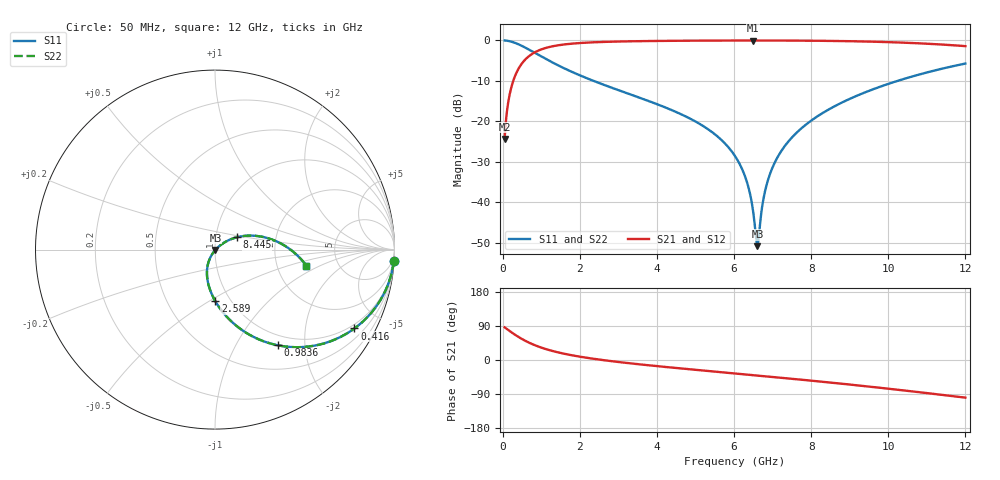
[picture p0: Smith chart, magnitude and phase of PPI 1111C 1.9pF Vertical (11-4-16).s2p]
# GHz S MA R 50
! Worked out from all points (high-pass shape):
!   1601 points, 50 MHz to 12 GHz, reference 50 ohm
!   highest |S21| = -0.03 dB at 6.496 GHz (marker M1); lowest = -24.4 dB at 50 MHz (marker M2)
!   |S21| within 3 dB of the highest: 818.2 MHz to end of sweep
!   lowest |S11| = -50.9 dB at 6.608 GHz (marker M3), VSWR 1.01, Z = 50.2 - j0.171 ohm
!   |S11| at or under -10 dB: 2.353 GHz to 10.24 GHz (7.891 GHz wide, 125 % of centre)
!   |S22| runs from -50.9 to 0.0 dB; largest |S21 - S12| = 0
!   S11 on the Smith chart (normalised r, x): 50 MHz: 1, -30; 416 MHz: 0.84, -3.62; 983.6 MHz: 0.84, -1.52; 2.589 GHz: 0.85, -0.53; 8.445 GHz: 1.26, +0.18; 12 GHz: 2.95, -0.72
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0.05  0.9982 -3.8  0.06055 86.2  0.06055 86.2  0.9982 -3.8
0.199375  0.9719 -14.9  0.2352 75.1  0.2352 75.1  0.9719 -14.9
0.4159687  0.8924 -29.5  0.4509 60.5  0.4509 60.5  0.8924 -29.5
0.6624375  0.7783 -43.2  0.6273 46.8  0.6273 46.8  0.7783 -43.2
0.9835938  0.6394 -56.6  0.768 33.4  0.768 33.4  0.6394 -56.6
1.446656  0.4889 -70.0  0.8712 19.9  0.8712 19.9  0.4889 -70.0
2.044156  0.3627 -81.8  0.9305 8.0  0.9305 8.0  0.3627 -81.8
2.589375  0.2864 -89.8  0.9565 -0.1  0.9565 -0.1  0.2864 -89.8
4.038312  0.1603 -105.8  0.9849 -16.5  0.9849 -16.5  0.1603 -105.8
5.293062  0.0817 -117.0  0.994 -28.7  0.994 -28.7  0.0817 -117.0
6.025  0.03716 -121.5  0.9964 -35.5  0.9964 -35.5  0.03716 -121.5
6.316281  0.0189 -119.9  0.9967 -38.2  0.9967 -38.2  0.0189 -119.9
6.495531  0.007667 -108.5  0.9968 -39.9  0.9968 -39.9  0.007667 -108.5
6.56275  0.003937 -84.6  0.9968 -40.5  0.9968 -40.5  0.003937 -84.6
6.607563  0.002856 -36.6  0.9968 -41.0  0.9968 -41.0  0.002856 -36.6
6.809219  0.01402 35.1  0.9966 -42.9  0.9966 -42.9  0.01402 35.1
7.033281  0.02928 39.1  0.9962 -45.0  0.9962 -45.0  0.02928 39.1
7.429125  0.05767 38.0  0.9947 -48.8  0.9947 -48.8  0.05767 38.0
8.019156  0.1034 33.4  0.9907 -54.6  0.9907 -54.6  0.1034 33.4
8.444875  0.139 29.5  0.9861 -59.0  0.9861 -59.0  0.139 29.5
10.01331  0.2912 13.2  0.9516 -75.9  0.9516 -75.9  0.2912 13.2
12  0.5172 -10.0  0.8495 -99.3  0.8495 -99.3  0.5172 -10.0
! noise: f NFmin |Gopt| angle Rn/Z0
0.05  0.0006383  0.9449  2.569  0.002591
1.372  0.00398  0.6935  11.23  0.002509
2.701  0.00642  0.6403  19.07  0.003283
4.031  0.008639  0.6158  26.84  0.00397
5.36  0.01081  0.6066  34.31  0.004665
6.682  0.013  0.608  41.33  0.005422
8.012  0.01534  0.6176  47.97  0.006307
9.341  0.01789  0.6338  54.19  0.007378
10.67  0.02074  0.6553  60.02  0.00872
12  0.024  0.681  65.52  0.01045
